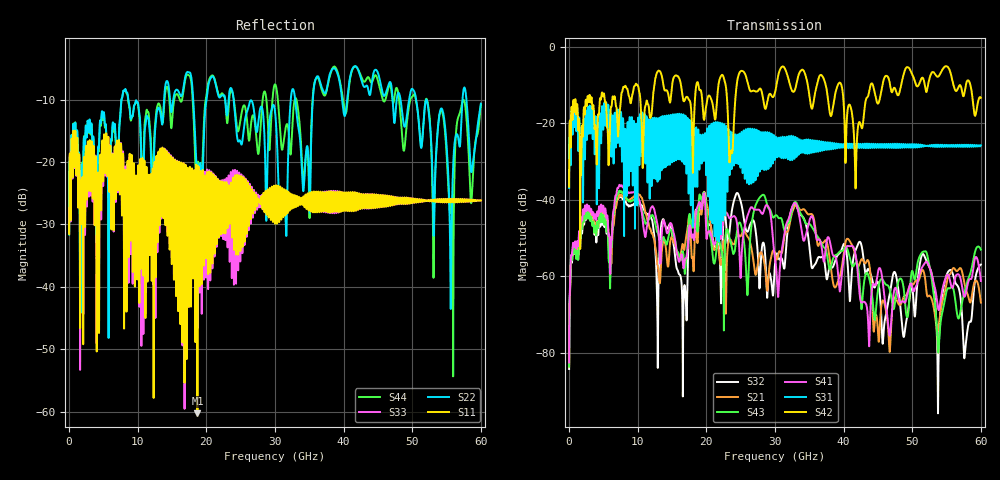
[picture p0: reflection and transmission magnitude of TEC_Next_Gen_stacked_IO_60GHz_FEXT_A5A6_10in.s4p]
!! CHANNEL DESCRIPTION:  Next Generation 28Gbps Press-fit Stacked I/O Connector
!!  with 10" 5-6-5 Megtron 6 Stripline trace on host side and 1.25" 7-5-7 Megtron 6 Microstrip trace on plug side
!! HOST PCB DESCRIPTION:  PCB thickness 3.425 mm
!!  26 Layer Board, 15 GND planes, 4 Layer route-out on Layers 7,11,17,21, 8mil stub on vias
!!  Pairs on following layers
!!  Layer 07 - A02A03 A14A15 D05D06
!!  Layer 11 - D020D3 C05C06 D14D15
!!  Layer 17 - C02C03 B05B06 C14C15
!!  Layer 21 - B02B03 A05A06 B14B15
!! CONNECTOR DESCRIPTION:  Next Generation 28Gbps Press-fit Stacked I/O Connector
!! PLUG-IN CARD DESCRIPTION:  PCB thickness 1mm thick
!!  6 Layer Board, 4 GND planes, 0.35 x 1.4mm mating pads
!!  Micro-strip diff traces referenced to GND plane 3mils down, 2nd GND plane 17mils from top of board
!!  PCB GND planes are symmetric
!! MODEL DESCRIPTION: TE Connectivity S-parameter model produced from Macro-model, Extracted .s4p FEXT (Victim B05B06 - Aggressor A05A06)
!! MODEL DATE: 5/15/2014 CR32f, FPR23
!! MODEL STATUS: Developmental
!! MODEL GEOMETRY: 4 Rows - Rows A, B, C, D. 3 pairs in each row, 12 total pairs
!! MODEL FREQUENCY RANGE: DC to 60 GHz in 10 MHz frequency steps
!! MODEL EDGE RATE LIMITATION: 8.33 ps (Using conservative 0.5/Fmax rule of thumb)
!! TIME-DOMAIN TRANSFORM CAUTIONS:
!! 1.) Do not simulate transient edge rates faster than the number listed above.  Edge
!!  rates faster than this number contain significant spectral content at frequencies
!!  above the model's highest frequency.
!! 2.) Even when simulating edge rates that are slower than the number listed above, be
!!  aware that the best time resolution possible with a direct iFFT is (1 / 2Fmax).
!!  As a result, time resolution is typically not adequate for most time-domain
!!  simulations unless tricks such as frequency-domain zero-padding and windowing are
!!  used to minimize leakage and aliasing.
!! 3.) Because the model has a uniform frequency step, a direct iFFT will result in an
!!  impulse that that has a time length given by either (1 / Fstep) or (1 / 2Fstep),
!!  depending on the transform being used.  Care has been taken in selecting the
!!  frequency step to ensure a settled impulse response for the model.  Therefore,
!!  convolution with the model's impulse response should present no issues.  However,
!!  if directly concatenating s-parameter models in the frequency domain a user must
!!  either interpolate necessary interim frequencies or complete impulse response
!!  zero-padding.  Impulse response zero-padding is more difficult, but more accurate.
!! PORT DEFINITIONS:
!! Port  1  ----->  Host A05		B05 Module <-----  Port  2
!! Port  3  ----->  Host A06		B06 Module <-----  Port  4
! Touchstone data
! Created: 29-Sep-2014 by IdEM R2011 (7.0.3)
# Hz S MA R 50
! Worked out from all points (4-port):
!   6000 points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, 10 MHz to 60 GHz, reference 50 ohm
!   strongest paths, dB at 10 MHz, 15.01 GHz, 30.01 GHz, 45.01 GHz, 60 GHz:
!     S42: -36.6, -10.1, -12.0, -14.9, -13.4
!     S31: -36.9, -25.4, -28.5, -25.5, -25.8
!     S41: -82.4, -46.8, -55.4, -58.8, -61.2
!     S43: -83.6, -48.3, -44.2, -63.5, -53.0
!     S21: -83.3, -49.8, -54.0, -74.6, -66.8
!     S32: -84.1, -48.9, -56.7, -61.6, -56.9
!   lowest |S11| = -60.3 dB at 18.7 GHz (marker M1), VSWR 1.00, Z = 50.1 - j0.00564 ohm
!   |S11| at or under -10 dB: start of sweep to end of sweep
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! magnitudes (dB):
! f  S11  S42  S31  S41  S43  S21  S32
! 10 MHz  -31.5  -36.6  -36.9  -82.4  -83.6  -83.3  -84.1
! 2.61 GHz  -26.0  -14.9  -24.1  -41.2  -42.8  -42.1  -42.9
! 16.84 GHz  -39.8  -14.0  -27.2  -55.9  -59.2  -52.6  -62.3
! 18.7 GHz  -60.3  -9.3  -31.6  -41.9  -48.3  -51.3  -45.0
! 51.85 GHz  -26.3  -10.3  -25.8  -56.5  -53.4  -60.3  -55.0
! 53.83 GHz  -26.3  -7.8  -25.8  -68.7  -79.5  -73.1  -82.1
! 60 GHz  -26.1  -13.4  -25.8  -61.2  -53.0  -66.8  -56.9
